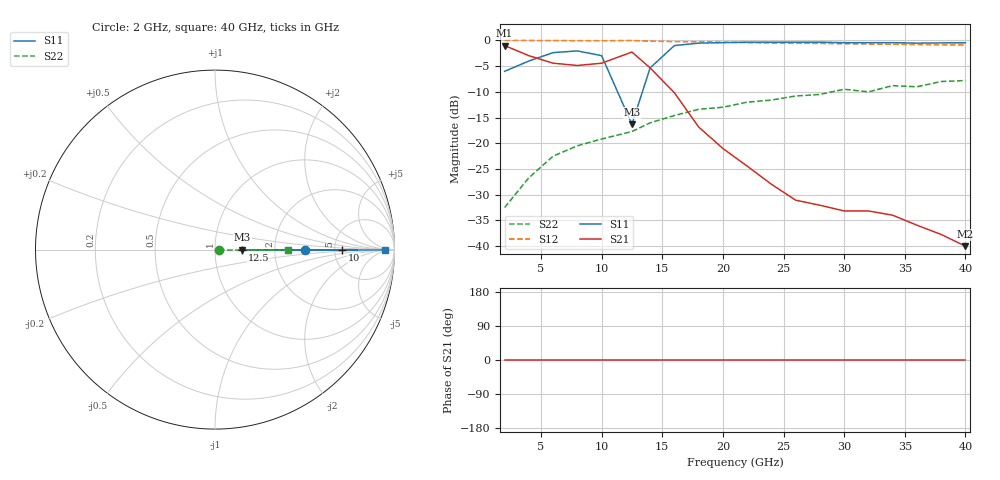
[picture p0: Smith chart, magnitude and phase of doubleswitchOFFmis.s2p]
# GHZ S MA R 50
!Output file by Shape3_28
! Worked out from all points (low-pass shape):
!   20 points, 2 GHz to 40 GHz, reference 50 ohm
!   highest |S21| = -1.01 dB at 2 GHz (marker M1); lowest = -40.0 dB at 40 GHz (marker M2)
!   |S21| within 3 dB of the highest: start of sweep to 5.419 GHz; 10.49 GHz to 13.35 GHz (2.858 GHz wide, 24 % of centre)
!   lowest |S11| = -16.3 dB at 12.5 GHz (marker M3), VSWR 1.36, Z = 68.1 + j0 ohm
!   |S11| at or under -10 dB: 11.32 GHz to 13.36 GHz (2.046 GHz wide, 16.6 % of centre)
!   |S22| runs from -32.5 to -7.8 dB; largest |S21 - S12| = 0.91
!   S11 on the Smith chart (normalised r, x): 2 GHz: 3.00, +0.00; 10 GHz: 5.90, +0.00; 12.5 GHz: 1.36, +0.00; 40 GHz: 37, +0
2  0.5 0.0  0.89 0.0  0.9979 0.0  0.0237 0.0
4  0.63 0.0  0.71 0.0  0.9972 0.0  0.0463 0.0
6  0.76 0.0  0.6 0.0  0.9951 0.0  0.075 0.0
8  0.79 0.0  0.57 0.0  0.9934 0.0  0.0944 0.0
10  0.71 0.0  0.6 0.0  0.9917 0.0  0.11 0.0
12.5  0.153 0.0  0.77 0.0  0.9965 0.0  0.13 0.0
14  0.54 0.0  0.54 0.0  0.983 0.0  0.158 0.0
16  0.89 0.0  0.31 0.0  0.973 0.0  0.186 0.0
18  0.94 0.0  0.144 0.0  0.968 0.0  0.214 0.0
20  0.95 0.0  0.089 0.0  0.96 0.0  0.224 0.0
22  0.96 0.0  0.06 0.0  0.95 0.0  0.251 0.0
24  0.96 0.0  0.04 0.0  0.944 0.0  0.263 0.0
26  0.96 0.0  0.028 0.0  0.938 0.0  0.288 0.0
28  0.96 0.0  0.025 0.0  0.9332 0.0  0.298 0.0
30  0.95 0.0  0.022 0.0  0.9279 0.0  0.335 0.0
32  0.95 0.0  0.022 0.0  0.9225 0.0  0.316 0.0
34  0.95 0.0  0.02 0.0  0.917 0.0  0.363 0.0
36  0.94 0.0  0.016 0.0  0.912 0.0  0.354 0.0
38  0.945 0.0  0.013 0.0  0.906 0.0  0.398 0.0
40  0.948 0.0  0.01 0.0  0.902 0.0  0.407 0.0
